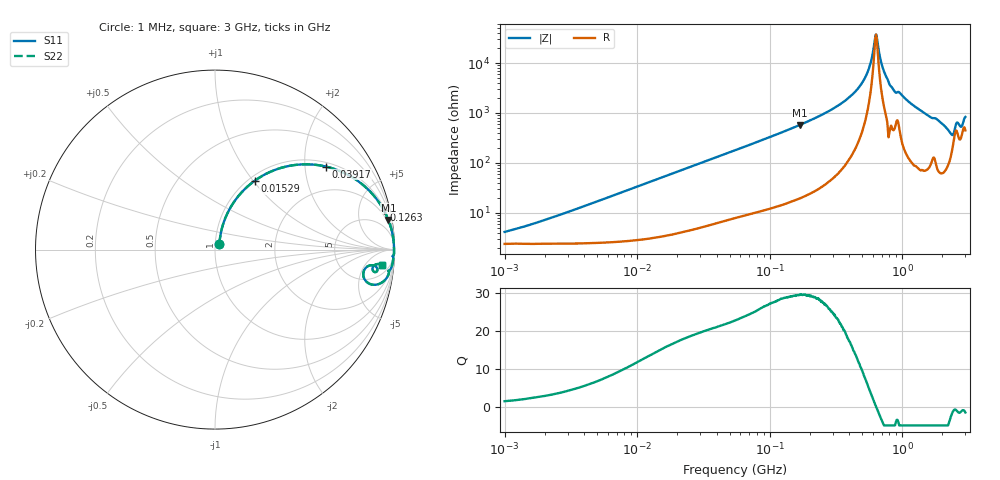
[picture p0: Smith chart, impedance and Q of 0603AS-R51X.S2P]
!s-Parameter Generated by FASTRON Sdn. Bhd.
!FASTRON P/N : 0603AS-R51X
!Keysight Technologies: E4991B_MY54100416_A.01.15
!Date created: Tue Oct 31 11:15:22 2023
!Version  : Rev01 Tue Oct 31 11:15:22 2023
!Data & Calibration Information:
!Freq	S11	S21	S12	S22
!PortZ  Port1:50+j0  Port2:50+j0
!When reading reference impedance value at option line is always used.
! Remarks : This data is being provided solely for informational purposes.
# Hz S dB R 50
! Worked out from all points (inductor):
!   1601 points, 1 MHz to 3 GHz, reference 50 ohm
!   read as one part in series: L = 535 nH near 2.15 MHz
!   highest Q = 29.6 at 169.7 MHz (marker M1), where L = 542 nH
!   self-resonance near 632.8 MHz
!   S11 on the Smith chart (normalised r, x): 1 MHz: 1.05, +0.07; 15.29 MHz: 1.07, +1.02; 39.17 MHz: 1.12, +2.57; 126.3 MHz: 1.29, +8.37; 3 GHz: 10, -14
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1000000  -27.87 53.0  -0.21 -1.9  -0.21 -1.9  -27.87 53.0
3804036  -18.00 72.1  -0.28 -7.1  -0.28 -7.1  -18.00 72.1
1.447069e7  -7.47 61.2  -1.13 -25.0  -1.13 -25.0  -7.47 61.2
1.528954e7  -7.09 60.1  -1.22 -26.2  -1.22 -26.2  -7.09 60.1
3.917023e7  -2.25 36.9  -4.43 -50.4  -4.43 -50.4  -2.25 36.9
5.477226e7  -1.34 28.6  -6.39 -58.9  -6.39 -58.9  -1.34 28.6
1.263238e8  -0.31 13.3  -12.74 -74.7  -12.74 -74.7  -0.31 13.3
1.697087e8  -0.18 9.7  -15.43 -78.3  -15.43 -78.3  -0.18 9.7
2.083556e8  -0.12 7.7  -17.47 -80.4  -17.47 -80.4  -0.12 7.7
3.402349e8  -0.05 3.8  -23.55 -83.6  -23.55 -83.6  -0.05 3.8
4.639993e8  -0.03 1.8  -29.83 -83.4  -29.83 -83.4  -0.03 1.8
5.528145e8  -0.02 0.8  -36.87 -78.6  -36.87 -78.6  -0.02 0.8
6.327845e8  -0.02 0.0  -51.40 -6.8  -51.40 -6.8  -0.02 0.0
6.520712e8  -0.02 -0.2  -48.35 45.6  -48.35 45.6  -0.02 -0.2
7.135306e8  -0.03 -0.7  -38.13 76.1  -38.13 76.1  -0.03 -0.7
7.925923e8  -0.02 -1.4  -32.22 83.7  -32.22 83.7  -0.02 -1.4
8.804142e8  -0.07 -2.1  -28.58 77.1  -28.58 77.1  -0.07 -2.1
1.921792e9  -0.21 -8.3  -16.75 76.3  -16.75 76.3  -0.21 -8.3
2.324278e9  -0.93 -12.6  -12.73 57.7  -12.73 57.7  -0.93 -12.6
2.581816e9  -0.92 -6.0  -17.02 41.6  -17.02 41.6  -0.92 -6.0
2.783064e9  -1.02 -7.7  -15.48 45.1  -15.48 45.1  -1.02 -7.7
3e9  -0.58 -5.4  -19.01 52.1  -19.01 52.1  -0.58 -5.4
